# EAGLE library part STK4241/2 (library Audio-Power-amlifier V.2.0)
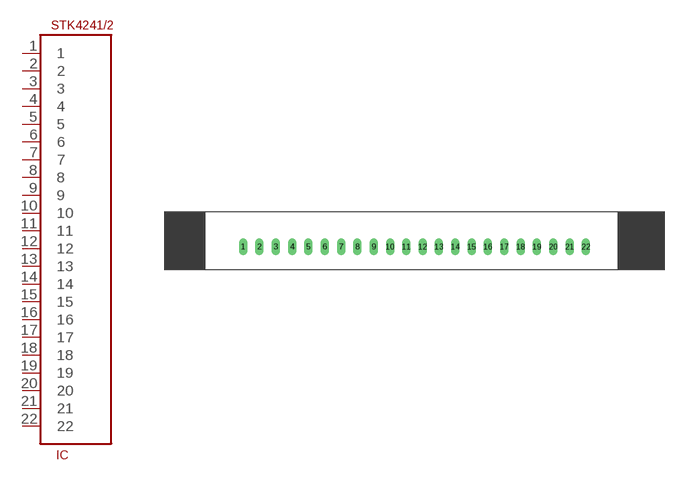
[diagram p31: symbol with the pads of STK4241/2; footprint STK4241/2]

Designator prefix IC

## STK4241/2  [STK4241/2]
1  1
2  2
3  3  in
4  4  in
5  5  pwr
6  6
7  7
8  8
9  9
10  10
11  11  pwr
12  12  out
13  13  pwr
14  14  pwr
15  15  out
16  16  pwr
17  17
18  18  pwr
19  19  in
20  20  in
21  21
22  22

## Footprint STK4241/2 (pad centres in mm)
drill 0.8 long: 1 -26.67,-1; 2 -24.13,-1; 3 -21.59,-1; 4 -19.05,-1; 5 -16.51,-1; 6 -13.97,-1; 7 -11.43,-1; 8 -8.89,-1; 9 -6.35,-1; 10 -3.81,-1; 11 -1.27,-1; 12 1.27,-1; 13 3.81,-1; 14 6.35,-1; 15 8.89,-1; 16 11.43,-1; 17 13.97,-1; 18 16.51,-1; 19 19.05,-1; 20 21.59,-1; 21 24.13,-1; 22 26.67,-1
